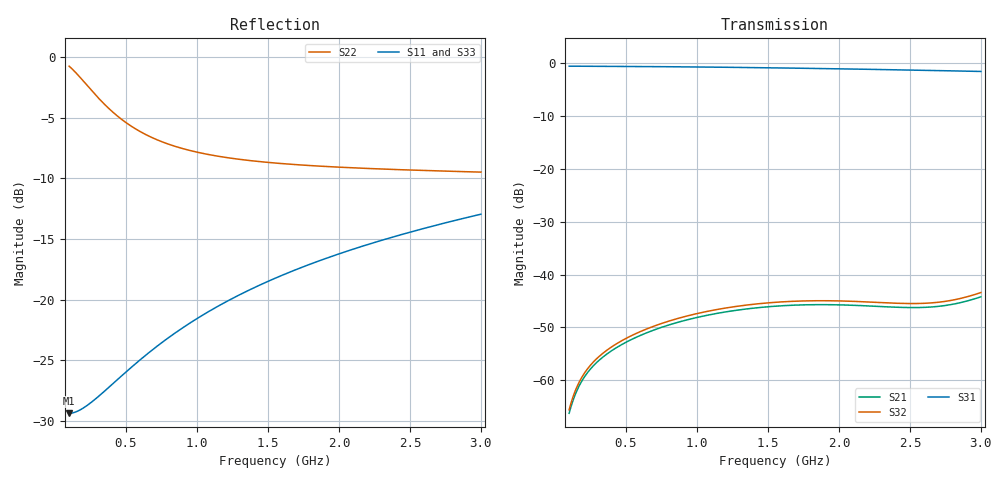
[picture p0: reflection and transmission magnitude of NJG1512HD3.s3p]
! Port1:P1 Port2:P2 Port3:PC
# hz S ma R 50
! 3 Port Network Data from SP1.SP block
! freq  magS11  angS11  magS12  angS12  magS13  angS13
!  magS21  angS21
!  magS22  angS22  magS23  angS23
!  magS31  angS31  magS32  angS32
!  magS33  angS33
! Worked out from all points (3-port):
!   291 points, 100 MHz to 3 GHz, reference 50 ohm
!   strongest paths, dB at 100 MHz, 820 MHz, 1.55 GHz, 2.28 GHz, 3 GHz:
!     S31: -0.5, -0.6, -0.8, -1.1, -1.5
!     S32: -65.6, -48.7, -45.3, -45.3, -43.4
!     S21: -66.3, -49.4, -46.0, -46.0, -44.2
!   lowest |S11| = -29.4 dB at 100 MHz (marker M1), VSWR 1.07, Z = 53.2 - j1.35 ohm
!   |S11| at or under -10 dB: start of sweep to end of sweep
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1e8  0.03403 -21.8  0.0004846 65.4  0.9426 -1.8
     0.0004846 65.4  0.9163 -15.4  0.0005228 66.4
     0.9426 -1.8  0.0005228 66.4  0.03397 -21.9
1.6e8  0.03474 -29.7  0.0008237 73.2  0.9413 -2.7
       0.0008237 73.2  0.8456 -22.2  0.0008935 74.0
       0.9413 -2.7  0.0008935 74.0  0.03475 -29.8
2.4e8  0.03715 -39.6  0.001227 74.0  0.9403 -3.9
       0.001227 74.0  0.7481 -28.7  0.001333 74.7
       0.9403 -3.9  0.001333 74.7  0.03729 -39.6
3.6e8  0.04252 -52.5  0.001742 73.8  0.9388 -5.8
       0.001742 73.8  0.6291 -33.9  0.001894 74.6
       0.9388 -5.8  0.001894 74.6  0.04288 -52.3
5e8  0.05034 -64.6  0.002281 73.9  0.9369 -8.0
     0.002281 73.9  0.5368 -36.2  0.002481 74.8
     0.9369 -8.0  0.002481 74.8  0.05096 -64.0
7.1e8  0.06368 -78.4  0.003025 74.1  0.9332 -11.3
       0.003025 74.1  0.4582 -36.8  0.003291 75.2
       0.9332 -11.3  0.003291 75.2  0.06467 -77.2
9.6e8  0.08075 -90.8  0.003809 73.9  0.9274 -15.3
       0.003809 73.9  0.4105 -36.9  0.004144 75.4
       0.9274 -15.3  0.004144 75.4  0.08213 -89.0
1.55e9  0.1225 -112.5  0.005012 74.2  0.9083 -24.4
        0.005012 74.2  0.3656 -39.4  0.005457 76.5
        0.9083 -24.4  0.005457 76.5  0.1245 -109.1
2.61e9  0.1974 -141.2  0.004893 104.3  0.8604 -40.4
        0.004893 104.3  0.3405 -51.4  0.005348 108.3
        0.8604 -40.4  0.005348 108.3  0.1993 -135.2
3e9  0.225 -150.2  0.006152 132.9  0.84 -46.2
     0.006152 132.9  0.3354 -57.6  0.006754 137.4
     0.84 -46.2  0.006754 137.4  0.2265 -143.4
